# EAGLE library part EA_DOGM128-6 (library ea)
ELECTRONIC ASSEMBLY GmbH EA DOGM128B-6 EA DOGM128E-6 EA DOGM128L-6 EA DOGM128S-6 EA DOGM128W-6
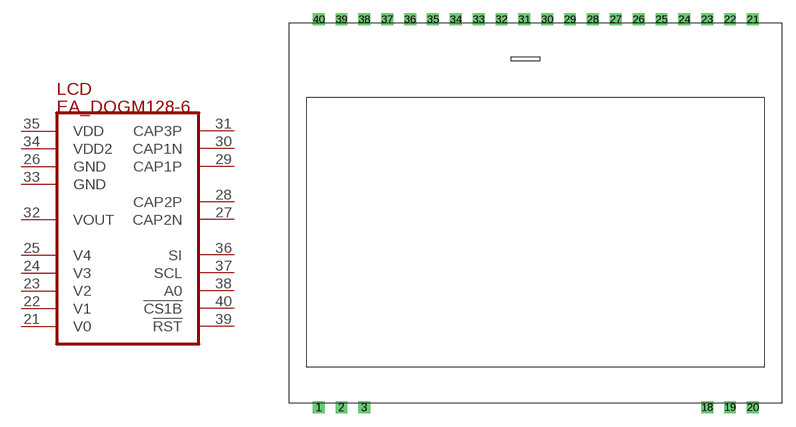
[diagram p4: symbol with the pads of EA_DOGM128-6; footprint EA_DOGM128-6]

Designator prefix LCD

## EA_DOGM128-6  [EA_DOGM128-6]
21  V0  in
22  V1  in
23  V2  pas
24  V3  pas
25  V4  pas
26  GND
27  CAP2N
28  CAP2P
29  CAP1P
30  CAP1N
31  CAP3P
32  VOUT  pas
33  GND
34  VDD2  pwr
35  VDD  pwr
36  SI
37  SCL  in
38  A0  in
39  !RST!  in
40  !CS1B!  in

## Footprint EA_DOGM128-6 (pad centres in mm)
EA DOGM128-6 Grafikdisplay COG 128x64 Pixel inkl.Kontroller Hersteller: ELECTRONIC ASSEMBLY GmbH http://www.lcd-module.de
drill 0.813 square: 1 0,0; 2 2.54,0; 3 5.08,0; 18 43.18,0; 19 45.72,0; 20 48.26,0; 21 48.26,43.18; 22 45.72,43.18; 23 43.18,43.18; 24 40.64,43.18; 25 38.1,43.18; 26 35.56,43.18; 27 33.02,43.18; 28 30.48,43.18; 29 27.94,43.18; 30 25.4,43.18; 31 22.86,43.18; 32 20.32,43.18; 33 17.78,43.18; 34 15.24,43.18; 35 12.7,43.18; 36 10.16,43.18; 37 7.62,43.18; 38 5.08,43.18; 39 2.54,43.18; 40 0,43.18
